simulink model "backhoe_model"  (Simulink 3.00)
settings: Solver=ode4  StartTime=0.0  StopTime=tfinal  FixedStep=T  RelTol=1e-3
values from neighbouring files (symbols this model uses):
  a1 = R(1,1)    [Jacobian.m]    (also in sub_static_vars.m = a(1))
  a2 = R(2,2)    [Jacobian.m]    (also in sub_static_vars.m = a(2))
  a3 = R(3,3)    [Jacobian.m]    (also in sub_static_vars.m = a(3))
  a4 = R(4,1)    [Jacobian.m]    (also in sub_static_vars.m = a(4))
  Ac = pi*(Dc.^2)/4    [cylinders.m]
  Ar = Ac-pi*(Dr.^2)/4    [cylinders.m]
  Cd = 2    [startup.m]
  dt = tfinal/N    (= 0.02)    [demo_trench.m]
  G1 = '0'    [sub_static_vars.m]    (also in symbolic_manip.m = G)
  G2 = char(G{2})    [sub_static_vars.m]    (also in symbolic_manip.m = G)
  G3 = char(G{3})    [sub_static_vars.m]    (also in symbolic_manip.m = G)
  G4 = char(G{4})    [sub_static_vars.m]    (also in symbolic_manip.m = G)
  Lcyl = [12.5*2 25 25.5 21.5]'    [cylinders.m]
  M11 = char(M{1})    [sub_static_vars.m]
  M12 = char(M{2})    [sub_static_vars.m]
  M13 = char(M{3})    [sub_static_vars.m]
  M14 = char(M{4})    [sub_static_vars.m]
  M21 = char(M{5})    [sub_static_vars.m]
  M22 = char(M{6})    [sub_static_vars.m]
  M23 = char(M{7})    [sub_static_vars.m]
  M24 = char(M{8})    [sub_static_vars.m]
  M31 = char(M{9})    [sub_static_vars.m]
  M32 = char(M{10})    [sub_static_vars.m]
  M33 = char(M{11})    [sub_static_vars.m]
  M34 = char(M{12})    [sub_static_vars.m]
  M41 = char(M{13})    [sub_static_vars.m]
  M42 = char(M{14})    [sub_static_vars.m]
  M43 = char(M{15})    [sub_static_vars.m]
  M44 = char(M{16})    [sub_static_vars.m]
  prelief = 2250    [backhoesim.m]
  pT = 0    [backhoesim.m]
  q0 = cyl_to_joint(yc0,R)    [backhoesim.m]
  qmax = cyl_to_joint([yclim(2,1) yclim(2,1) yclim(1,2) yclim(1,3) yclim(1,4)],R)    [backhoesim.m]    (also in demo_trench.m = [1.5708    1.0907    6.1403    6.5025])
  qmin = cyl_to_joint([yclim(1,1) yclim(1,1) yclim(2,2) yclim(2,3) yclim(2,4)],R)    [backhoesim.m]    (also in demo_trench.m = [-1.5708   -0.8529    3.6469    4.1089])
  QP = 33.11    [backhoesim.m]
  R1A = R(1,5)    [cyl_to_joint.m]    (also in dimensions.m = sqrt(R0N^2+(R01-RAN)^2); joint_to_cyl.m; SFr2taur.m; Sjoint_to_cyl.m)
  R1B = R(2,4)    [cyl_to_joint.m]    (also in dimensions.m = 35.875; joint_to_cyl.m; SFr2taur.m; Sjoint_to_cyl.m)
  R2C = R(2,3)    [cyl_to_joint.m]    (also in dimensions.m = 36; joint_to_cyl.m; SFr2taur.m; Sjoint_to_cyl.m)
  R2D = R(3,1)    [cyl_to_joint.m]    (also in dimensions.m = 9.875; joint_to_cyl.m; SFr2taur.m; Sjoint_to_cyl.m)
  R3F = R(3,5)-R(3,7)    [cyl_to_joint.m]    (also in dimensions.m = 4.5; joint_to_cyl.m; SFr2taur.m = R(3,8); Sjoint_to_cyl.m)
  R3G = R(4,2)    [cyl_to_joint.m]    (also in dimensions.m = 5.5; joint_to_cyl.m; SFr2taur.m; Sjoint_to_cyl.m)
  REF = R(3,6)    [cyl_to_joint.m]    (also in dimensions.m = 30.77; joint_to_cyl.m; SFr2taur.m; Sjoint_to_cyl.m)
  RFH = R(4,4)    [cyl_to_joint.m]    (also in dimensions.m = 9.5; joint_to_cyl.m; SFr2taur.m; Sjoint_to_cyl.m)
  RGH = R(4,5)    [cyl_to_joint.m]    (also in dimensions.m = 9.5; joint_to_cyl.m; SFr2taur.m; Sjoint_to_cyl.m)
  T = 0.001    [startup.m]
  T01A = R(1,12)    [cyl_to_joint.m]    (also in dimensions.m = atan(R0N/(R01-RAN)); joint_to_cyl.m; Sjoint_to_cyl.m)
  T12C = R(2,13)    [cyl_to_joint.m]    (also in dimensions.m = acos((R12^2+R2C^2-R1C^2)/(2*R12*R2C)); joint_to_cyl.m; Sjoint_to_cyl.m)
  T23D = acos((R23^2+R3D^2-R2D^2)/(2*R23*R3D))    [cyl_to_joint.m]    (also in dimensions.m; joint_to_cyl.m = R(3,14); SFr2taur.m = R(3,14); Sjoint_to_cyl.m = R(3,14))
  TB12 = R(2,12)    [cyl_to_joint.m]    (also in dimensions.m = acos((R1B^2+R12^2-R2B^2)/(2*R1B*R12)); joint_to_cyl.m; SFr2taur.m; Sjoint_to_cyl.m)
  TD23 = R(3,12)    [cyl_to_joint.m]    (also in dimensions.m = acos((R2D^2+R23^2-R3D^2)/(2*R2D*R23)); joint_to_cyl.m; SFr2taur.m; Sjoint_to_cyl.m)
  TDFE = R(3,13)    [cyl_to_joint.m]    (also in dimensions.m = acos((RDF^2+REF^2-RDE^2)/(2*RDF*REF)); joint_to_cyl.m; SFr2taur.m; Sjoint_to_cyl.m)
  TG34 = R(4,12)    [cyl_to_joint.m]    (also in dimensions.m = acos((R3G^2+R34^2-R4G^2)/(2*R3G*R34)); joint_to_cyl.m; SFr2taur.m; Sjoint_to_cyl.m)
  V1 = char(V{1})    [sub_static_vars.m]    (also in symbolic_manip.m = V)
  V2 = char(V{2})    [sub_static_vars.m]    (also in symbolic_manip.m = V)
  V3 = char(V{3})    [sub_static_vars.m]    (also in symbolic_manip.m = V)
  V4 = char(V{4})    [sub_static_vars.m]    (also in symbolic_manip.m = V)
  yc0 = [21.587 21.587 28.9 45.27 36.195]'    [backhoesim.m]
undefined symbols (not defined in the file or in its folder): Cc, Cr, den, K1, kd, Kr, num, pc0, pr0, td, wn, zeta
libraries: simulink3 x2
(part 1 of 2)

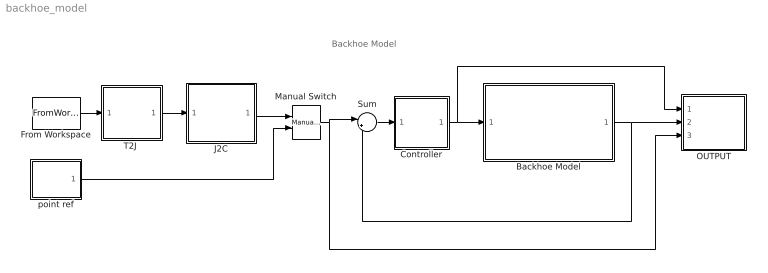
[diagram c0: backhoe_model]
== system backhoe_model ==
  note: Backhoe Model
  Backhoe Model : Subsystem
  Controller : Subsystem
  From Workspace : FromWorkspace  VariableName=traj  SampleTime=0  HoldFinalValue=off
  J2C : Subsystem
  Manual Switch : simulink3/Nonlinear/Manual Switch  sw=1  action=0
  OUTPUT : Subsystem
  Sum : Sum  Inputs=|+-  SaturateOnIntegerOverflow=on
  "T2J " : Subsystem
  point ref : Subsystem
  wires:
  Sum/1 -> Controller/1(e)
  Backhoe Model/1(yc_th) -> Sum/2, OUTPUT/2(yc_th)
  Controller/1(Us) -> Backhoe Model/1(Us), OUTPUT/1(Us)
  Manual Switch/1 -> Sum/1, OUTPUT/3(ycdes)
  J2C/1(ycdes) -> Manual Switch/1
  "T2J "/1(qdes) -> J2C/1(qdes)
  From Workspace/1 -> "T2J "/1(ybdes)
  point ref/1(ycdes) -> Manual Switch/2

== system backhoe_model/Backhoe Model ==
  note: Note: input voltages need to range between (3,9) [V]
  note: predicted position sensor measurements
  Us : Inport  Port=1  PortWidth=-1  SampleTime=-1  DataType=auto
  Backhoe Dynamics : Subsystem
  Hoses & Cylinders : Subsystem
  Mux : Mux  Inputs=2
  PVG32 Valve Bank : Subsystem
  Selector : Selector  Elements=[3 4 5]  InputPortWidth=5
  Subsystem : Subsystem
  Terminator5 : Terminator
  Terminator6 : Terminator
  pump flow rate : Constant  Value=QP
  soil wrench : Constant  Value=[0 0 0 0 0 0]
  tank pressure : Constant  Value=pT
  yc_th : Outport  Port=1
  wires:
  Backhoe Dynamics/3(yc) -> Hoses & Cylinders/3(yc), Selector/1
  Backhoe Dynamics/2(yed) -> Terminator5/1
  soil wrench/1 -> Backhoe Dynamics/2(We)
  [pcyl] -> PVG32 Valve Bank/2(pcyl)
  pump flow rate/1 -> PVG32 Valve Bank/3(QP)
  tank pressure/1 -> PVG32 Valve Bank/4(pT)
  Hoses & Cylinders/2(Fr) -> Backhoe Dynamics/1(Fr)
  Backhoe Dynamics/1(ye) -> Terminator6/1
  Us/1 -> PVG32 Valve Bank/1(Us)
  Selector/1 -> Mux/2
  Backhoe Dynamics/4(q1) -> Mux/1
  Hoses & Cylinders/1(pcyl) -> [pcyl], Subsystem/1(pcyl1)
  Mux/1 -> yc_th/1
  PVG32 Valve Bank/1(Qc) -> Hoses & Cylinders/1(Qc)
  PVG32 Valve Bank/2(Qr) -> Hoses & Cylinders/2(Qr)

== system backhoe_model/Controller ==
  note: Controller
  e : Inport  Port=1  PortWidth=-1  SampleTime=-1  DataType=auto
  Anti-deadband : Subsystem
  D-Gain : Gain  Gain=[0 0 0 0]  SaturateOnIntegerOverflow=on
  Derivative : Derivative
  I-Gain : Gain  Gain=[0 0 0 0]  SaturateOnIntegerOverflow=on
  Integrator : Integrator  ExternalReset=none  InitialConditionSource=internal  InitialCondition=0  LimitOutput=on  UpperSaturationLimit=1  LowerSaturationLimit=-1  ShowSaturationPort=off  ShowStatePort=off  AbsoluteTolerance=auto
  Manual Switch : simulink3/Nonlinear/Manual Switch  sw=1  action=0
  P-Gain : Gain  Gain=[0.8 0.8 0.8 0.8]  SaturateOnIntegerOverflow=on
  Standard : Subsystem
  Sum : Sum  Inputs=+++  SaturateOnIntegerOverflow=on
  voltage limits : Saturate  UpperLimit=9  LowerLimit=3
  Us : Outport  Port=1
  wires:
  e/1 -> P-Gain/1, I-Gain/1, D-Gain/1
  D-Gain/1 -> Derivative/1
  Integrator/1 -> Sum/2
  I-Gain/1 -> Integrator/1
  P-Gain/1 -> Sum/1
  Derivative/1 -> Sum/3
  Sum/1 -> Anti-deadband/1(us), Standard/1(us)
  Standard/1(Us) -> Manual Switch/1
  Manual Switch/1 -> voltage limits/1
  voltage limits/1 -> Us/1
  Anti-deadband/1(Us) -> Manual Switch/2

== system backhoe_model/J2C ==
  note: Joint Space -> Cylinder Space Transformation
  note: Swing Cylinders
  qdes : Inport  Port=1  PortWidth=-1  SampleTime=-1  DataType=auto
  Boom cylinder : Subsystem
  Bucket cylinder : Subsystem
  Demux : Demux  Outputs=4
  Mux : Mux  Inputs=4
  Stick cylinder : Subsystem
  overswing  protection : Saturate  UpperLimit=pi/3  LowerLimit=-pi/2
  ycdes : Outport  Port=1
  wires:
  qdes/1 -> Demux/1
  Mux/1 -> ycdes/1
  Demux/2 -> Boom cylinder/1(q2)
  Boom cylinder/1(yc3) -> Mux/2
  Demux/3 -> Stick cylinder/1(q3)
  Stick cylinder/1(yc4) -> Mux/3
  Demux/4 -> Bucket cylinder/1(q4)
  Bucket cylinder/1(yc5) -> Mux/4
  Demux/1 -> overswing  protection/1
  overswing  protection/1 -> Mux/1

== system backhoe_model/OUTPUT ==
  Us : Inport  Port=1  PortWidth=-1  SampleTime=-1  DataType=auto
  yc_th : Inport  Port=2  PortWidth=-1  SampleTime=-1  DataType=auto
  ycdes : Inport  Port=3  PortWidth=-1  SampleTime=-1  DataType=auto
  Clock : Clock
  Demux : Demux  Outputs=4
  Demux1 : Demux  Outputs=4
  Mux : Mux  Inputs=4
  Mux{1..4} (4 alike) : Mux  Inputs=2
  To Workspace : ToWorkspace  VariableName=data_th  SampleTime=-1  SaveFormat=Matrix
  Us1 : Scope
  yc : Scope  NumInputPorts=4
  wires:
  Mux/1 -> To Workspace/1
  Clock/1 -> Mux/1
  Us/1 -> Mux/2, Us1/1
  yc_th/1 -> Mux/3, Demux/1
  Mux1/1 -> yc/1
  Mux2/1 -> yc/2
  Mux3/1 -> yc/3
  Mux4/1 -> yc/4
  Demux1/1 -> Mux1/1
  Demux/1 -> Mux1/2
  Demux1/2 -> Mux2/1
  Demux/2 -> Mux2/2
  Demux1/3 -> Mux3/1
  Demux/3 -> Mux3/2
  Demux1/4 -> Mux4/1
  Demux/4 -> Mux4/2
  ycdes/1 -> Demux1/1, Mux/4

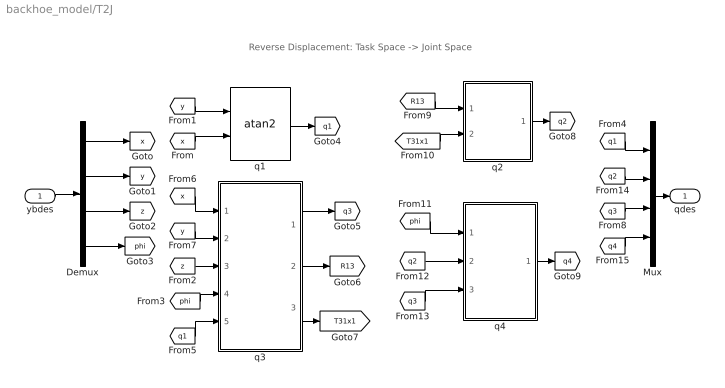
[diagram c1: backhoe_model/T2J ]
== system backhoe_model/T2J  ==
  note: Reverse Displacement: Task Space -> Joint Space
  ybdes : Inport  Port=1  PortWidth=-1  SampleTime=-1  DataType=auto
  Demux : Demux  Outputs=4
  Mux : Mux  Inputs=4
  q1 : Trigonometry  Operator=atan2  OutputSignalType=auto
  q2 : Subsystem
  q3 : Subsystem
  q4 : Subsystem
  qdes : Outport  Port=1
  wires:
  [x] -> q3/1(x)
  [y] -> q3/2(y)
  [z] -> q3/3(z)
  [phi] -> q3/4(phi)
  [q1] -> q3/5(q1)
  q3/1(q3) -> [q3]
  q3/2(R13) -> [R13]
  [y] -> q1/1
  q1/1 -> [q1]
  q3/3(T31x1) -> [T31x1]
  [R13] -> q2/1(R13)
  [T31x1] -> q2/2(T31x1)
  [q3] -> q4/3(q3)
  [q2] -> q4/2(q2)
  [phi] -> q4/1(phi)
  q2/1(q2) -> [q2]
  q4/1(q4) -> [q4]
  Mux/1 -> qdes/1
  [q1] -> Mux/1
  [q3] -> Mux/3
  [q2] -> Mux/2
  [q4] -> Mux/4
  ybdes/1 -> Demux/1
  Demux/1 -> [x]
  Demux/2 -> [y]
  Demux/3 -> [z]
  Demux/4 -> [phi]
  [x] -> q1/2

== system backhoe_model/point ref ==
  Boom : Sin  Amplitude=0  Frequency=1  Phase=0  SampleTime=0
  Bucket : Sin  Amplitude=0  Frequency=1  Phase=0  SampleTime=0
  Mux : Mux  Inputs=4
  Stick : Sin  Amplitude=0  Frequency=1  Phase=0  SampleTime=0
  Sum : Sum  Inputs=|++  SaturateOnIntegerOverflow=on
  Swing : Sin  Amplitude=0.3  Frequency=0.7  Phase=0  SampleTime=0
  initial cylinder lengths : Constant  Value=[q0(1) yc0(3) yc0(4) yc0(5)]
  ycdes : Outport  Port=1
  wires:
  Swing/1 -> Mux/1
  Boom/1 -> Mux/2
  Bucket/1 -> Mux/4
  Stick/1 -> Mux/3
  Mux/1 -> Sum/1
  initial cylinder lengths/1 -> Sum/2
  Sum/1 -> ycdes/1

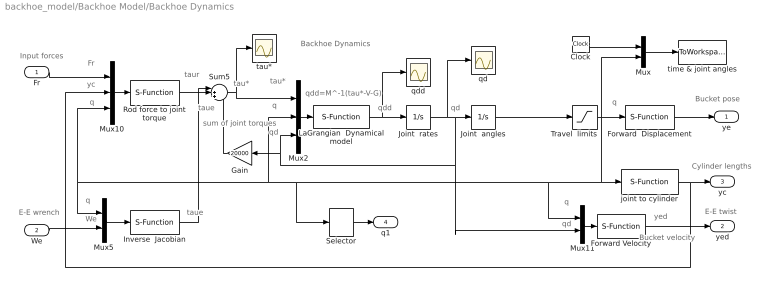
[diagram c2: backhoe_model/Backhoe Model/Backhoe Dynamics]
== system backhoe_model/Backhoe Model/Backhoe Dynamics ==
  note: taur
  note: tau*
  note: qdd
  note: qd
  note: qdd=M^-1(tau*-V-G)
  note: q
  note: q
  note: taue
  note: taue
  note: Bucket velocity
  note: yed
  note: qd
  note: q
  note: qd
  note: Fr
  note: q
  note: tau*
  note: sum of joint torques
  note: yc
  note: q
  note: We
  note: Backhoe Dynamics
  note: E-E wrench
  note: Input forces
  note: Bucket pose
  note: Cylinder lengths
  note: E-E twist
  Fr : Inport  Port=1  PortWidth=-1  SampleTime=-1  DataType=auto
  We : Inport  Port=2  PortWidth=-1  SampleTime=-1  DataType=auto
  Clock : Clock
  Forward Velocity : S-Function  FunctionName=SFvel  Parameters=R  PortCounts=[]  SFunctionModules=''
  Forward  Displacement : S-Function  FunctionName=SFdisp  Parameters=a  PortCounts=[]  SFunctionModules=''
  Gain : Gain  Orientation=left  Gain=20000  SaturateOnIntegerOverflow=on
  Inverse  Jacobian : S-Function  FunctionName=SRtorque  Parameters=R  PortCounts=[]  SFunctionModules=''
  Joint  angles : Integrator  ExternalReset=none  InitialConditionSource=internal  InitialCondition=q0  LimitOutput=off  UpperSaturationLimit=inf  LowerSaturationLimit=-inf  ShowSaturationPort=off  ShowStatePort=off  AbsoluteTolerance=auto
  Joint  rates : Integrator  ExternalReset=none  InitialConditionSource=internal  InitialCondition=0  LimitOutput=off  UpperSaturationLimit=inf  LowerSaturationLimit=-inf  ShowSaturationPort=off  ShowStatePort=off  AbsoluteTolerance=auto
  LaGrangian  Dynamical model : S-Function  FunctionName=SLaGrange  Parameters=M11,M12,M13,M14,M21,M22,M23,M24,M31,M32,M33,M34,M41,M42,M43,M44,V1,V2,V3,V4,G1,G2,G3,G4  PortCounts=[]  SFunctionModules=''
  Mux : Mux  Inputs=2
  Mux10 : Mux  Inputs=3
  Mux11 : Mux  Inputs=2
  Mux2 : Mux  Inputs=3
  Mux5 : Mux  Inputs=2
  Rod force to joint torque : S-Function  FunctionName=SFr2taur  Parameters=R  PortCounts=[]  SFunctionModules=''
  Selector : Selector  Elements=1  InputPortWidth=4
  Sum5 : Sum  Inputs=|++-  SaturateOnIntegerOverflow=on
  Travel  limits : Saturate  UpperLimit=qmax  LowerLimit=qmin
  joint to cylinder : S-Function  FunctionName=Sjoint_to_cyl  Parameters=R, yc0  PortCounts=[]  SFunctionModules=''
  qd : Scope
  qdd : Scope
  tau* : Scope
  time & joint angles : ToWorkspace  VariableName=tq  SampleTime=-1  SaveFormat=Matrix
  ye : Outport  Port=1
  yed : Outport  Port=2
  yc : Outport  Port=3
  q1 : Outport  Port=4
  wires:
  Mux2/1 -> LaGrangian  Dynamical model/1
  Mux10/1 -> Rod force to joint torque/1
  Rod force to joint torque/1 -> Sum5/1
  Mux5/1 -> Inverse  Jacobian/1
  Inverse  Jacobian/1 -> Sum5/2
  We/1 -> Mux5/2
  Selector/1 -> q1/1
  Sum5/1 -> Mux2/1, tau*/1
  Fr/1 -> Mux10/1
  LaGrangian  Dynamical model/1 -> Joint  rates/1, qdd/1
  Joint  rates/1 -> Mux11/2, Mux2/3, Gain/1, Joint  angles/1, qd/1
  Clock/1 -> Mux/1
  Travel  limits/1 -> Forward  Displacement/1, Mux11/1, Mux2/2, Mux5/1, Mux10/3, Selector/1, joint to cylinder/1, Mux/2
  Mux11/1 -> Forward Velocity/1
  joint to cylinder/1 -> yc/1, Mux10/2
  Forward Velocity/1 -> yed/1
  Forward  Displacement/1 -> ye/1
  Mux/1 -> time & joint angles/1
  Joint  angles/1 -> Travel  limits/1
  Gain/1 -> Sum5/3

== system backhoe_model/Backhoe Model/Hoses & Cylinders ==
  note: DVc
  note: DVr
  note: pc
  note: cap pressures
  note: pr
  note: rod pressures
  note: pressure forces on rods
  note: yc
  note: yc
  note: Hoses and Cylinders
  Qc : Inport  Port=1  PortWidth=-1  SampleTime=-1  DataType=auto
  Qr : Inport  Port=2  PortWidth=-1  SampleTime=-1  DataType=auto
  yc : Inport  Port=3  PortWidth=-1  SampleTime=-1  DataType=auto
  Cap areas : Gain  Gain=Ac  SaturateOnIntegerOverflow=on
  Cap-side compressible  volume : S-Function  FunctionName=SCcap  Parameters=Ac,Cc,yc0,pc0  PortCounts=[]  SFunctionModules=''
  DVcDVr : Scope  NumInputPorts=2
  Fr1 : Scope
  Integrator : Integrator  ExternalReset=none  InitialConditionSource=internal  InitialCondition=0  LimitOutput=on  UpperSaturationLimit=Lcyl.*Ac  LowerSaturationLimit=-Lcyl.*Ac  ShowSaturationPort=off  ShowStatePort=off  AbsoluteTolerance=auto
  Integrator1 : Integrator  ExternalReset=none  InitialConditionSource=internal  InitialCondition=0  LimitOutput=on  UpperSaturationLimit=Lcyl.*Ar  LowerSaturationLimit=-Lcyl.*Ar  ShowSaturationPort=off  ShowStatePort=off  AbsoluteTolerance=auto
  Mux : Mux  Inputs=2
  Mux7 : Mux  Inputs=2
  Mux8 : Mux  Inputs=2
  QcycQr : Scope  NumInputPorts=3
  Rod areas : Gain  Gain=Ar  SaturateOnIntegerOverflow=on
  Rod-side compressible volume : S-Function  FunctionName=SCrod  Parameters=Ar,Cr,yc0,pr0  PortCounts=[]  SFunctionModules=''
  Sum4 : Sum  Inputs=+|-  SaturateOnIntegerOverflow=on
  anti-cavitation : Saturate  UpperLimit=prelief  LowerLimit=0
  anti-cavitation1 : Saturate  UpperLimit=prelief  LowerLimit=0
  pcyl : Outport  Port=1
  Fr : Outport  Port=2
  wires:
  Cap-side compressible  volume/1 -> anti-cavitation/1
  Rod-side compressible volume/1 -> anti-cavitation1/1
  Cap areas/1 -> Sum4/1
  Mux/1 -> pcyl/1
  anti-cavitation/1 -> Cap areas/1, Mux/1
  anti-cavitation1/1 -> Rod areas/1, Mux/2
  yc/1 -> Mux8/2, Mux7/2, QcycQr/2
  Rod areas/1 -> Sum4/2
  Qr/1 -> Integrator1/1, QcycQr/3
  Qc/1 -> Integrator/1, QcycQr/1
  Sum4/1 -> Fr/1, Fr1/1
  Mux7/1 -> Cap-side compressible  volume/1
  Mux8/1 -> Rod-side compressible volume/1
  Integrator/1 -> Mux7/1, DVcDVr/1
  Integrator1/1 -> Mux8/1, DVcDVr/2

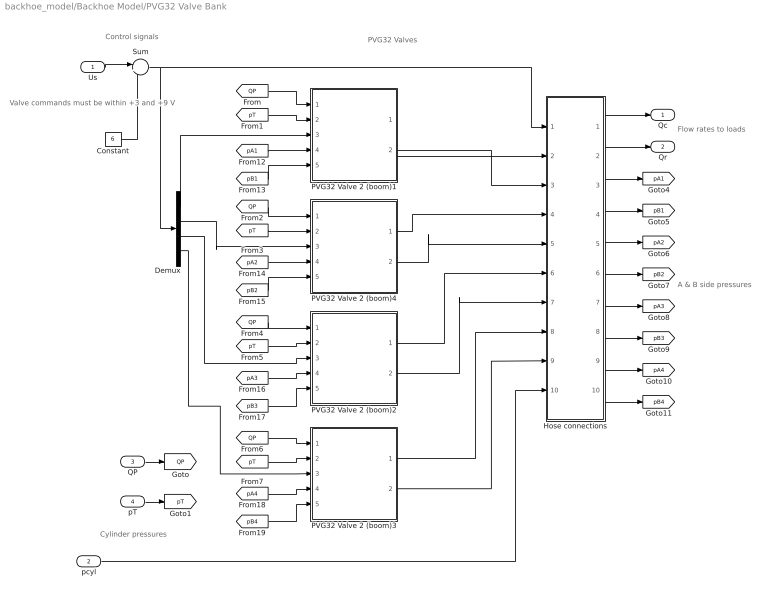
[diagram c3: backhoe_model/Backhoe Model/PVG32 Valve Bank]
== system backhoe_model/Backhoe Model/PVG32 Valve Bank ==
  note: Flow rates to loads
  note: Control signals
  note: PVG32 Valves
  note: Cylinder pressures
  note: A & B side pressures
  note: Valve commands must be within +3 and +9 V
  Us : Inport  Port=1  PortWidth=-1  SampleTime=-1  DataType=auto
  pcyl : Inport  Port=2  PortWidth=-1  SampleTime=-1  DataType=auto
  QP : Inport  Port=3  PortWidth=-1  SampleTime=-1  DataType=auto
  pT : Inport  Port=4  PortWidth=-1  SampleTime=-1  DataType=auto
  Constant : Constant  Value=6
  Demux : Demux  Outputs=4
  Hose connections : Subsystem
  PVG32 Valve 2 (boom)1 : Subsystem
  PVG32 Valve 2 (boom)2 : Subsystem
  PVG32 Valve 2 (boom)3 : Subsystem
  PVG32 Valve 2 (boom)4 : Subsystem
  Sum : Sum  Inputs=|+-  SaturateOnIntegerOverflow=on
  Qc : Outport  Port=1
  Qr : Outport  Port=2
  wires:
  Hose connections/1(Qc) -> Qc/1
  Hose connections/2(Qr) -> Qr/1
  Hose connections/3(pA1) -> [pA1]
  Hose connections/4(pB1) -> [pB1]
  Hose connections/5(pA2) -> [pA2]
  Hose connections/6(pB2) -> [pB2]
  Hose connections/7(pA3) -> [pA3]
  Hose connections/8(pB3) -> [pB3]
  Hose connections/9(pA4) -> [pA4]
  Hose connections/10(pB4) -> [pB4]
  pcyl/1 -> Hose connections/10(pcyl)
  Demux/1 -> PVG32 Valve 2 (boom)1/3(Us)
  [QP] -> PVG32 Valve 2 (boom)1/1(QP)
  [pT] -> PVG32 Valve 2 (boom)1/2(pT)
  [pA1] -> PVG32 Valve 2 (boom)1/4(pA)
  [pB1] -> PVG32 Valve 2 (boom)1/5(pB)
  Demux/2 -> PVG32 Valve 2 (boom)4/3(Us)
  [pT] -> PVG32 Valve 2 (boom)4/2(pT)
  [QP] -> PVG32 Valve 2 (boom)4/1(QP)
  Demux/3 -> PVG32 Valve 2 (boom)2/3(Us)
  [pA2] -> PVG32 Valve 2 (boom)4/4(pA)
  [pB2] -> PVG32 Valve 2 (boom)4/5(pB)
  [pT] -> PVG32 Valve 2 (boom)2/2(pT)
  [QP] -> PVG32 Valve 2 (boom)2/1(QP)
  [pA3] -> PVG32 Valve 2 (boom)2/4(pA)
  [pB3] -> PVG32 Valve 2 (boom)2/5(pB)
  Demux/4 -> PVG32 Valve 2 (boom)3/3(Us)
  QP/1 -> [QP]
  pT/1 -> [pT]
  [QP] -> PVG32 Valve 2 (boom)3/1(QP)
  [pT] -> PVG32 Valve 2 (boom)3/2(pT)
  [pA4] -> PVG32 Valve 2 (boom)3/4(pA)
  [pB4] -> PVG32 Valve 2 (boom)3/5(pB)
  PVG32 Valve 2 (boom)1/1(QA) -> Hose connections/2(QA1)
  PVG32 Valve 2 (boom)1/2(QB) -> Hose connections/3(QB1)
  PVG32 Valve 2 (boom)4/1(QA) -> Hose connections/4(QA2)
  PVG32 Valve 2 (boom)4/2(QB) -> Hose connections/5(QB2)
  PVG32 Valve 2 (boom)2/1(QA) -> Hose connections/6(QA3)
  PVG32 Valve 2 (boom)2/2(QB) -> Hose connections/7(QB3)
  PVG32 Valve 2 (boom)3/1(QA) -> Hose connections/8(QA4)
  PVG32 Valve 2 (boom)3/2(QB) -> Hose connections/9(QB4)
  Us/1 -> Sum/1
  Constant/1 -> Sum/2
  Sum/1 -> Demux/1, Hose connections/1(Us)

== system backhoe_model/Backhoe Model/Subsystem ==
  pcyl1 : Inport  Port=1  PortWidth=-1  SampleTime=-1  DataType=auto
  Selector : Selector  Elements=[1 5]  InputPortWidth=8
  Selector1 : Selector  Elements=[2 6]  InputPortWidth=8
  Selector2 : Selector  Elements=[3 7]  InputPortWidth=8
  Selector3 : Selector  Elements=[4 8]  InputPortWidth=8
  To Workspace : ToWorkspace  VariableName=pcyl  SampleTime=-1  SaveFormat=Matrix
  pcyl : Scope  NumInputPorts=4
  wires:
  pcyl1/1 -> To Workspace/1, Selector3/1, Selector2/1, Selector/1, Selector1/1
  Selector/1 -> pcyl/1
  Selector1/1 -> pcyl/2
  Selector2/1 -> pcyl/3
  Selector3/1 -> pcyl/4

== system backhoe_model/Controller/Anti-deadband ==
  us : Inport  Port=1  PortWidth=-1  SampleTime=-1  DataType=auto
  Demux : Demux  Outputs=4
  Look-Up Table{,1..3} (4 alike) : Lookup  InputValues=[-1 0.02 0.02 1]  OutputValues=[3 5.45 6.55 9]
  Mux : Mux  Inputs=4
  Saturation : Saturate  UpperLimit=9  LowerLimit=3
  Us : Outport  Port=1
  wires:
  Demux/1 -> Look-Up Table/1
  Demux/2 -> Look-Up Table1/1
  Demux/3 -> Look-Up Table2/1
  Demux/4 -> Look-Up Table3/1
  Look-Up Table/1 -> Mux/1
  us/1 -> Demux/1
  Mux/1 -> Saturation/1
  Saturation/1 -> Us/1
  Look-Up Table1/1 -> Mux/2
  Look-Up Table2/1 -> Mux/3
  Look-Up Table3/1 -> Mux/4

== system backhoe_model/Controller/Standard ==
  us : Inport  Port=1  PortWidth=-1  SampleTime=-1  DataType=auto
  Gain : Gain  Gain=[10 3 3 1.5]  SaturateOnIntegerOverflow=on
  Sum1 : Sum  Inputs=|++  SaturateOnIntegerOverflow=on
  neutral : Constant  Value=6
  Us : Outport  Port=1
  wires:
  us/1 -> Gain/1
  neutral/1 -> Sum1/2
  Gain/1 -> Sum1/1
  Sum1/1 -> Us/1

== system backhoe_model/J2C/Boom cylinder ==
  q2 : Inport  Port=1  PortWidth=-1  SampleTime=-1  DataType=auto
  Constant : Constant  Value=pi
  Constant1 : Constant  Value=T01A
  Constant2 : Constant  Value=TB12
  CosineLawB : Subsystem
  Sum : Sum  Inputs=+---  SaturateOnIntegerOverflow=on
  yc3 : Outport  Port=1
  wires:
  Constant/1 -> Sum/1
  Constant1/1 -> Sum/2
  Sum/1 -> CosineLawB/1(TA1B)
  CosineLawB/1(yc3) -> yc3/1
  q2/1 -> Sum/3
  Constant2/1 -> Sum/4

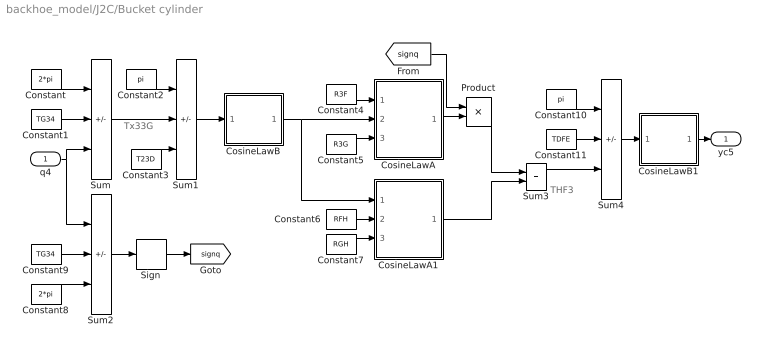
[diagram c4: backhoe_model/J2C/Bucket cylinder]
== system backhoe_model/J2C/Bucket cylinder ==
  note: Tx33G
  note: THF3
  q4 : Inport  Port=1  PortWidth=-1  SampleTime=-1  DataType=auto
  Constant : Constant  Value=2*pi
  Constant1 : Constant  Value=TG34
  Constant10 : Constant  Value=pi
  Constant11 : Constant  Value=TDFE
  Constant2 : Constant  Value=pi
  Constant3 : Constant  Value=T23D
  Constant4 : Constant  Value=R3F
  Constant5 : Constant  Value=R3G
  Constant6 : Constant  Value=RFH
  Constant7 : Constant  Value=RGH
  Constant8 : Constant  Value=2*pi
  Constant9 : Constant  Value=TG34
  CosineLawA : Subsystem
  CosineLawA1 : Subsystem
  CosineLawB : Subsystem
  CosineLawB1 : Subsystem
  Product : Product  Inputs=2  SaturateOnIntegerOverflow=on
  Sign : Signum
  Sum : Sum  Inputs=+--  SaturateOnIntegerOverflow=on
  Sum1 : Sum  Inputs=+-+  SaturateOnIntegerOverflow=on
  Sum2 : Sum  Inputs=++-  SaturateOnIntegerOverflow=on
  Sum3 : Sum  Inputs=++  SaturateOnIntegerOverflow=on
  Sum4 : Sum  Inputs=+--  SaturateOnIntegerOverflow=on
  yc5 : Outport  Port=1
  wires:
  Constant/1 -> Sum/1
  Constant1/1 -> Sum/2
  Sum/1 -> Sum1/2
  Constant2/1 -> Sum1/1
  Sum1/1 -> CosineLawB/1(TG3F)
  CosineLawB/1(rFG) -> CosineLawA/2(r2), CosineLawA1/1(r1)
  Constant4/1 -> CosineLawA/1(r1)
  Constant5/1 -> CosineLawA/3(r3)
  Constant6/1 -> CosineLawA1/2(r2)
  Constant7/1 -> CosineLawA1/3(r3)
  Constant9/1 -> Sum2/2
  Sum2/1 -> Sign/1
  [signq] -> Product/1
  CosineLawA/1(T3FG) -> Product/2
  Sign/1 -> [signq]
  Product/1 -> Sum3/1
  CosineLawA1/1(THFG) -> Sum3/2
  Constant10/1 -> Sum4/1
  Constant11/1 -> Sum4/2
  Sum4/1 -> CosineLawB1/1(TEFH)
  CosineLawB1/1(yc5) -> yc5/1
  q4/1 -> Sum2/1, Sum/3
  Constant3/1 -> Sum1/3
  Sum3/1 -> Sum4/3
  Constant8/1 -> Sum2/3

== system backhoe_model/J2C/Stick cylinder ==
  q3 : Inport  Port=1  PortWidth=-1  SampleTime=-1  DataType=auto
  Constant : Constant  Value=pi
  Constant1 : Constant  Value=TD23
  Constant2 : Constant  Value=T12C
  CosineLawB : Subsystem
  Sum : Sum  Inputs=+---  SaturateOnIntegerOverflow=on
  yc4 : Outport  Port=1
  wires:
  Constant/1 -> Sum/1
  Constant1/1 -> Sum/2
  Sum/1 -> CosineLawB/1(TC2D)
  CosineLawB/1(yc4) -> yc4/1
  q3/1 -> Sum/3
  Constant2/1 -> Sum/4

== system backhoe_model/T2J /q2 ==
  note: T213
  R13 : Inport  Port=1  PortWidth=-1  SampleTime=-1  DataType=auto
  T31x1 : Inport  Port=2  PortWidth=-1  SampleTime=-1  DataType=auto
  CosineLawA : Subsystem
  Sum : Sum  Inputs=|++  SaturateOnIntegerOverflow=on
  a2 : Constant  Value=a2
  a3 : Constant  Value=a3
  q2 : Outport  Port=1
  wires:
  a2/1 -> CosineLawA/1(r1)
  a3/1 -> CosineLawA/3(r3)
  CosineLawA/1(theta) -> Sum/1
  Sum/1 -> q2/1
  R13/1 -> CosineLawA/2(r2)
  T31x1/1 -> Sum/2

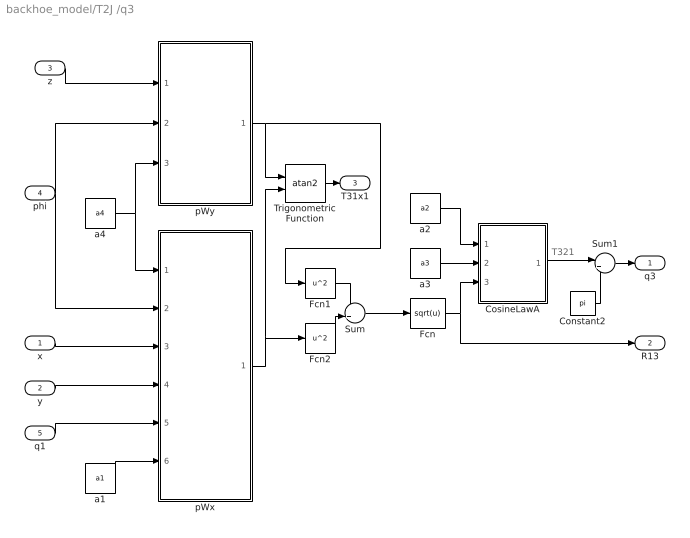
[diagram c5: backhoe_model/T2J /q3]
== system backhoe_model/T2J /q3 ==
  note: T321
  x : Inport  Port=1  PortWidth=-1  SampleTime=-1  DataType=auto
  y : Inport  Port=2  PortWidth=-1  SampleTime=-1  DataType=auto
  z : Inport  Port=3  PortWidth=-1  SampleTime=-1  DataType=auto
  phi : Inport  Port=4  PortWidth=-1  SampleTime=-1  DataType=auto
  q1 : Inport  Port=5  PortWidth=-1  SampleTime=-1  DataType=auto
  Constant2 : Constant  Value=pi
  CosineLawA : Subsystem
  Fcn : Fcn  Expr=sqrt(u)
  Fcn1 : Fcn  Expr=u^2
  Fcn2 : Fcn  Expr=u^2
  Sum : Sum  Inputs=++  SaturateOnIntegerOverflow=on
  Sum1 : Sum  Inputs=|++  SaturateOnIntegerOverflow=on
  Trigonometric Function : Trigonometry  Operator=atan2  OutputSignalType=auto
  a1 : Constant  Value=a1
  a2 : Constant  Value=a2
  a3 : Constant  Value=a3
  a4 : Constant  Value=a4
  pWx : Subsystem
  pWy : Subsystem
  q3 : Outport  Port=1
  R13 : Outport  Port=2
  T31x1 : Outport  Port=3
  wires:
  a1/1 -> pWx/6(a1)
  q1/1 -> pWx/5(q1)
  y/1 -> pWx/4(y)
  x/1 -> pWx/3(x)
  a4/1 -> pWx/1(a4), pWy/3(a4)
  z/1 -> pWy/1(z)
  phi/1 -> pWx/2(phi), pWy/2(phi)
  pWy/1(pWy) -> Fcn1/1, Trigonometric Function/1
  Trigonometric Function/1 -> T31x1/1
  Fcn1/1 -> Sum/1
  Fcn2/1 -> Sum/2
  Sum/1 -> Fcn/1
  a3/1 -> CosineLawA/2(r2)
  a2/1 -> CosineLawA/1(r1)
  Fcn/1 -> CosineLawA/3(r3), R13/1
  Sum1/1 -> q3/1
  Constant2/1 -> Sum1/2
  CosineLawA/1(theta) -> Sum1/1
  pWx/1(pWx) -> Fcn2/1, Trigonometric Function/2

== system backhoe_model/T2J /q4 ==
  phi : Inport  Port=1  PortWidth=-1  SampleTime=-1  DataType=auto
  q2 : Inport  Port=2  PortWidth=-1  SampleTime=-1  DataType=auto
  q3 : Inport  Port=3  PortWidth=-1  SampleTime=-1  DataType=auto
  Constant : Constant  Value=3*pi
  Sum : Sum  Inputs=+--+  SaturateOnIntegerOverflow=on
  q4 : Outport  Port=1
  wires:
  phi/1 -> Sum/1
  q2/1 -> Sum/2
  Sum/1 -> q4/1
  q3/1 -> Sum/3
  Constant/1 -> Sum/4

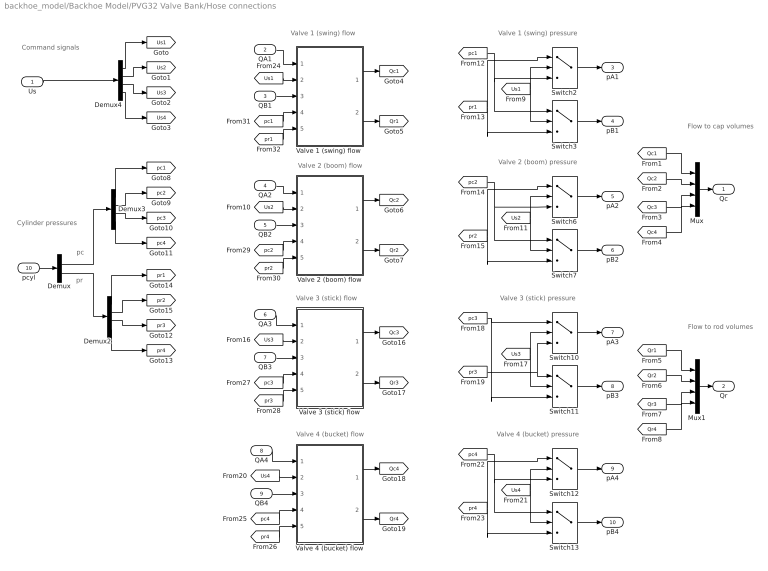
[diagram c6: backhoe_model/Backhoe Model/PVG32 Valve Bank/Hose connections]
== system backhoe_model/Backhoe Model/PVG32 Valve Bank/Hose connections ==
  note: pc
  note: pr
  note: Valve 1 (swing) flow
  note: Valve 1 (swing) pressure
  note: Valve 2 (boom) pressure
  note: Valve 3 (stick) flow
  note: Valve 3 (stick) pressure
  note: Valve 4 (bucket) flow
  note: Valve 4 (bucket) pressure
  note: Command signals
  note: Cylinder pressures
  note: Flow to rod volumes
  note: Flow to cap volumes
  note: Valve 2 (boom) flow
  Us : Inport  Port=1  PortWidth=-1  SampleTime=-1  DataType=auto
  QA1 : Inport  Port=2  PortWidth=-1  SampleTime=-1  DataType=auto
  QB1 : Inport  Port=3  PortWidth=-1  SampleTime=-1  DataType=auto
  QA2 : Inport  Port=4  PortWidth=-1  SampleTime=-1  DataType=auto
  QB2 : Inport  Port=5  PortWidth=-1  SampleTime=-1  DataType=auto
  QA3 : Inport  Port=6  PortWidth=-1  SampleTime=-1  DataType=auto
  QB3 : Inport  Port=7  PortWidth=-1  SampleTime=-1  DataType=auto
  QA4 : Inport  Port=8  PortWidth=-1  SampleTime=-1  DataType=auto
  QB4 : Inport  Port=9  PortWidth=-1  SampleTime=-1  DataType=auto
  pcyl : Inport  Port=10  PortWidth=-1  SampleTime=-1  DataType=auto
  Demux : Demux  Outputs=2
  Demux2 : Demux  Outputs=4
  Demux3 : Demux  Outputs=4
  Demux4 : Demux  Outputs=4
  Mux : Mux  Inputs=4
  Mux1 : Mux  Inputs=4
  Switch{2..3,6..7,10..13} (8 alike) : Switch  Threshold=0
  "Valve 1 (swing) flow " : Subsystem
  Valve 2 (boom) flow : Subsystem
  Valve 3 (stick) flow : Subsystem
  Valve 4 (bucket) flow : Subsystem
  Qc : Outport  Port=1
  Qr : Outport  Port=2
  pA1 : Outport  Port=3
  pB1 : Outport  Port=4
  pA2 : Outport  Port=5
  pB2 : Outport  Port=6
  pA3 : Outport  Port=7
  pB3 : Outport  Port=8
  pA4 : Outport  Port=9
  pB4 : Outport  Port=10
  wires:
  [Us1] -> Switch2/2, Switch3/2
  Switch2/1 -> pA1/1
  Switch3/1 -> pB1/1
  Demux3/1 -> [pc1]
  Demux3/2 -> [pc2]
  Demux3/3 -> [pc3]
  Demux3/4 -> [pc4]
  Demux2/1 -> [pr1]
  Demux2/2 -> [pr2]
  Demux2/3 -> [pr3]
  Demux2/4 -> [pr4]
  Demux4/1 -> [Us1]
  Demux4/2 -> [Us2]
  Demux4/3 -> [Us3]
  Demux4/4 -> [Us4]
  pcyl/1 -> Demux/1
  [pc1] -> Switch2/3, Switch3/1
  [pr1] -> Switch2/1, Switch3/3
  Demux/2 -> Demux2/1
  Demux/1 -> Demux3/1
  [Qc1] -> Mux/1
  [Qc2] -> Mux/2
  [Qc3] -> Mux/3
  [Qc4] -> Mux/4
  [Qr1] -> Mux1/1
  [Qr2] -> Mux1/2
  [Qr3] -> Mux1/3
  [Qr4] -> Mux1/4
  Mux/1 -> Qc/1
  Mux1/1 -> Qr/1
  Switch13/1 -> pB4/1
  Switch12/1 -> pA4/1
  [Us4] -> Switch12/2, Switch13/2
  [pc4] -> Switch12/3, Switch13/1
  [pr4] -> Switch13/3, Switch12/1
  Valve 4 (bucket) flow/1(Qc) -> [Qc4]
  Valve 4 (bucket) flow/2(Qr) -> [Qr4]
  QB4/1 -> Valve 4 (bucket) flow/3(QB)
  [Us4] -> Valve 4 (bucket) flow/2(Us)
  QA4/1 -> Valve 4 (bucket) flow/1(QA)
  [pc4] -> Valve 4 (bucket) flow/4(pc4)
  [pr4] -> Valve 4 (bucket) flow/5(pr4)
  [pr1] -> "Valve 1 (swing) flow "/5(pr1)
  [pc1] -> "Valve 1 (swing) flow "/4(pc1)
  QB1/1 -> "Valve 1 (swing) flow "/3(QB)
  [Us1] -> "Valve 1 (swing) flow "/2(Us)
  QA1/1 -> "Valve 1 (swing) flow "/1(QA)
  "Valve 1 (swing) flow "/1(Qc) -> [Qc1]
  "Valve 1 (swing) flow "/2(Qr) -> [Qr1]
  [Us2] -> Switch6/2, Switch7/2
  Switch6/1 -> pA2/1
  Switch7/1 -> pB2/1
  [pc2] -> Switch6/3, Switch7/1
  [pr2] -> Switch6/1, Switch7/3
  [pc2] -> Valve 2 (boom) flow/4(pc2)
  [pr2] -> Valve 2 (boom) flow/5(pr2)
  Valve 2 (boom) flow/1(Qc) -> [Qc2]
  Valve 2 (boom) flow/2(Qr) -> [Qr2]
  [Us2] -> Valve 2 (boom) flow/2(Us)
  QA2/1 -> Valve 2 (boom) flow/1(QA)
  QB2/1 -> Valve 2 (boom) flow/3(QB)
  Switch11/1 -> pB3/1
  Switch10/1 -> pA3/1
  [pr3] -> Switch11/1, Switch10/3
  [pc3] -> Switch10/1, Switch11/3
  [Us3] -> Switch10/2, Switch11/2
  Valve 3 (stick) flow/2(Qr) -> [Qr3]
  Valve 3 (stick) flow/1(Qc) -> [Qc3]
  [Us3] -> Valve 3 (stick) flow/2(Us)
  QA3/1 -> Valve 3 (stick) flow/1(QA)
  QB3/1 -> Valve 3 (stick) flow/3(QB)
  [pc3] -> Valve 3 (stick) flow/4(pc3)
  [pr3] -> Valve 3 (stick) flow/5(pr3)
  Us/1 -> Demux4/1

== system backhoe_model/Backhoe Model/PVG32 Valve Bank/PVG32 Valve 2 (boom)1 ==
  note: flow to load
  note: flow through relief valve
  QP : Inport  Port=1  PortWidth=-1  SampleTime=-1  DataType=auto
  pT : Inport  Port=2  PortWidth=-1  SampleTime=-1  DataType=auto
  Us : Inport  Port=3  PortWidth=-1  SampleTime=-1  DataType=auto
  pA : Inport  Port=4  PortWidth=-1  SampleTime=-1  DataType=auto
  pB : Inport  Port=5  PortWidth=-1  SampleTime=-1  DataType=auto
  Crossover relief : Subsystem  Orientation=left
  Dead Zone : DeadZone  LowerValue=-.5  UpperValue=.5
  Flow direction : Subsystem
  Input Averaging : Subsystem
  Product : Product  Inputs=2  SaturateOnIntegerOverflow=on
  SS gain : Subsystem
  Sum : Sum  Inputs=|+-  SaturateOnIntegerOverflow=on
  Terminator : Terminator
  Terminator2 : Terminator
  Time  Delay : TransportDelay  DelayTime=td  InitialInput=0  BufferSize=2048
  Valve dynamics : TransferFcn  Numerator=num  Denominator=den
  pump limits : Saturate  UpperLimit=QP  LowerLimit=-QP
  QA : Outport  Port=1
  QB : Outport  Port=2
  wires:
  pB/1 -> Flow direction/4(pB)
  pA/1 -> Flow direction/3(pA)
  pT/1 -> Terminator2/1
  Time  Delay/1 -> Valve dynamics/1
  Us/1 -> Dead Zone/1
  Dead Zone/1 -> Time  Delay/1, Flow direction/1(Us), Input Averaging/1(Us)
  Valve dynamics/1 -> Product/1
  Input Averaging/1(Ubar) -> SS gain/1(Ubar)
  SS gain/1(Kv) -> Product/2
  Product/1 -> Sum/1, Crossover relief/3(Q)
  Crossover relief/1(Qrelief) -> Sum/2
  QP/1 -> Terminator/1
  Sum/1 -> pump limits/1
  Flow direction/1(QA) -> QA/1
  Flow direction/2(QB) -> QB/1
  Flow direction/4(pR) -> Crossover relief/1(pR)
  Flow direction/3(pL) -> Crossover relief/2(pL)
  pump limits/1 -> Flow direction/2(Q)

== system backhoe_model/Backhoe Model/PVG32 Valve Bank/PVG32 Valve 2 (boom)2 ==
  note: flow to load
  note: flow through relief valve
  QP : Inport  Port=1  PortWidth=-1  SampleTime=-1  DataType=auto
  pT : Inport  Port=2  PortWidth=-1  SampleTime=-1  DataType=auto
  Us : Inport  Port=3  PortWidth=-1  SampleTime=-1  DataType=auto
  pA : Inport  Port=4  PortWidth=-1  SampleTime=-1  DataType=auto
  pB : Inport  Port=5  PortWidth=-1  SampleTime=-1  DataType=auto
  Crossover relief : Subsystem  Orientation=left
  Dead Zone : DeadZone  LowerValue=-.5  UpperValue=.5
  Flow direction : Subsystem
  Input Averaging : Subsystem
  Product : Product  Inputs=2  SaturateOnIntegerOverflow=on
  SS gain : Subsystem
  Sum : Sum  Inputs=|+-  SaturateOnIntegerOverflow=on
  Terminator : Terminator
  Terminator2 : Terminator
  Time  Delay : TransportDelay  DelayTime=td  InitialInput=0  BufferSize=2048
  Valve dynamics : TransferFcn  Numerator=num  Denominator=den
  pump limits : Saturate  UpperLimit=QP  LowerLimit=-QP
  QA : Outport  Port=1
  QB : Outport  Port=2
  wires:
  pB/1 -> Flow direction/4(pB)
  pA/1 -> Flow direction/3(pA)
  pT/1 -> Terminator2/1
  Time  Delay/1 -> Valve dynamics/1
  Us/1 -> Dead Zone/1
  Dead Zone/1 -> Time  Delay/1, Flow direction/1(Us), Input Averaging/1(Us)
  Valve dynamics/1 -> Product/1
  Input Averaging/1(Ubar) -> SS gain/1(Ubar)
  SS gain/1(Kv) -> Product/2
  Product/1 -> Sum/1, Crossover relief/3(Q)
  Crossover relief/1(Qrelief) -> Sum/2
  QP/1 -> Terminator/1
  Sum/1 -> pump limits/1
  Flow direction/1(QA) -> QA/1
  Flow direction/2(QB) -> QB/1
  Flow direction/4(pR) -> Crossover relief/1(pR)
  Flow direction/3(pL) -> Crossover relief/2(pL)
  pump limits/1 -> Flow direction/2(Q)

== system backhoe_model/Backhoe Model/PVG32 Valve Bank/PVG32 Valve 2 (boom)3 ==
  note: flow to load
  note: flow through relief valve
  QP : Inport  Port=1  PortWidth=-1  SampleTime=-1  DataType=auto
  pT : Inport  Port=2  PortWidth=-1  SampleTime=-1  DataType=auto
  Us : Inport  Port=3  PortWidth=-1  SampleTime=-1  DataType=auto
  pA : Inport  Port=4  PortWidth=-1  SampleTime=-1  DataType=auto
  pB : Inport  Port=5  PortWidth=-1  SampleTime=-1  DataType=auto
  Crossover relief : Subsystem  Orientation=left
  Dead Zone : DeadZone  LowerValue=-.5  UpperValue=.5
  Flow direction : Subsystem
  Input Averaging : Subsystem
  Product : Product  Inputs=2  SaturateOnIntegerOverflow=on
  SS gain : Subsystem
  Sum : Sum  Inputs=|+-  SaturateOnIntegerOverflow=on
  Terminator : Terminator
  Terminator2 : Terminator
  Time  Delay : TransportDelay  DelayTime=td  InitialInput=0  BufferSize=2048
  Valve dynamics : TransferFcn  Numerator=num  Denominator=den
  pump limits : Saturate  UpperLimit=QP  LowerLimit=-QP
  QA : Outport  Port=1
  QB : Outport  Port=2
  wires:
  pB/1 -> Flow direction/4(pB)
  pA/1 -> Flow direction/3(pA)
  pT/1 -> Terminator2/1
  Time  Delay/1 -> Valve dynamics/1
  Us/1 -> Dead Zone/1
  Dead Zone/1 -> Time  Delay/1, Flow direction/1(Us), Input Averaging/1(Us)
  Valve dynamics/1 -> Product/1
  Input Averaging/1(Ubar) -> SS gain/1(Ubar)
  SS gain/1(Kv) -> Product/2
  Product/1 -> Sum/1, Crossover relief/3(Q)
  Crossover relief/1(Qrelief) -> Sum/2
  QP/1 -> Terminator/1
  Sum/1 -> pump limits/1
  Flow direction/1(QA) -> QA/1
  Flow direction/2(QB) -> QB/1
  Flow direction/4(pR) -> Crossover relief/1(pR)
  Flow direction/3(pL) -> Crossover relief/2(pL)
  pump limits/1 -> Flow direction/2(Q)

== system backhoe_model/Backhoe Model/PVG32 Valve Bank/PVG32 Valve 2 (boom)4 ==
  note: flow to load
  note: flow through relief valve
  QP : Inport  Port=1  PortWidth=-1  SampleTime=-1  DataType=auto
  pT : Inport  Port=2  PortWidth=-1  SampleTime=-1  DataType=auto
  Us : Inport  Port=3  PortWidth=-1  SampleTime=-1  DataType=auto
  pA : Inport  Port=4  PortWidth=-1  SampleTime=-1  DataType=auto
  pB : Inport  Port=5  PortWidth=-1  SampleTime=-1  DataType=auto
  Crossover relief : Subsystem  Orientation=left
  Dead Zone : DeadZone  LowerValue=-.5  UpperValue=.5
  Flow direction : Subsystem
  Input Averaging : Subsystem
  Product : Product  Inputs=2  SaturateOnIntegerOverflow=on
  SS gain : Subsystem
  Sum : Sum  Inputs=|+-  SaturateOnIntegerOverflow=on
  Terminator : Terminator
  Terminator2 : Terminator
  Time  Delay : TransportDelay  DelayTime=td  InitialInput=0  BufferSize=2048
  Valve dynamics : TransferFcn  Numerator=num  Denominator=den
  pump limits : Saturate  UpperLimit=QP  LowerLimit=-QP
  QA : Outport  Port=1
  QB : Outport  Port=2
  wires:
  pB/1 -> Flow direction/4(pB)
  pA/1 -> Flow direction/3(pA)
  pT/1 -> Terminator2/1
  Time  Delay/1 -> Valve dynamics/1
  Us/1 -> Dead Zone/1
  Dead Zone/1 -> Time  Delay/1, Flow direction/1(Us), Input Averaging/1(Us)
  Valve dynamics/1 -> Product/1
  Input Averaging/1(Ubar) -> SS gain/1(Ubar)
  SS gain/1(Kv) -> Product/2
  Product/1 -> Sum/1, Crossover relief/3(Q)
  Crossover relief/1(Qrelief) -> Sum/2
  QP/1 -> Terminator/1
  Sum/1 -> pump limits/1
  Flow direction/1(QA) -> QA/1
  Flow direction/2(QB) -> QB/1
  Flow direction/4(pR) -> Crossover relief/1(pR)
  Flow direction/3(pL) -> Crossover relief/2(pL)
  pump limits/1 -> Flow direction/2(Q)

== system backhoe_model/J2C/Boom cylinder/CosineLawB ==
  TA1B : Inport  Port=1  PortWidth=-1  SampleTime=-1  DataType=auto
  Constant : Constant  Value=2
  Product : Product  Inputs=4  SaturateOnIntegerOverflow=on
  Sum2 : Sum  Inputs=-++  SaturateOnIntegerOverflow=on
  cosine : Trigonometry  Operator=cos  OutputSignalType=auto
  rA : Constant  Value=R1A
  rB : Constant  Value=R1B
  sqr : Fcn  Expr=u^2
  sqr1 : Fcn  Expr=u^2
  sqrt : Fcn  Expr=sqrt(u)
  yc3 : Outport  Port=1
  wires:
  rA/1 -> sqr/1, Product/2
  sqr1/1 -> Sum2/3
  Constant/1 -> Product/1
  sqr/1 -> Sum2/2
  Product/1 -> Sum2/1
  Sum2/1 -> sqrt/1
  TA1B/1 -> cosine/1
  sqrt/1 -> yc3/1
  rB/1 -> sqr1/1, [rB]
  [rB] -> Product/3
  cosine/1 -> Product/4

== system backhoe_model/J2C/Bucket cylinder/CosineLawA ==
  r1 : Inport  Port=1  PortWidth=-1  SampleTime=-1  DataType=auto
  r2 : Inport  Port=2  PortWidth=-1  SampleTime=-1  DataType=auto
  r3 : Inport  Port=3  PortWidth=-1  SampleTime=-1  DataType=auto
  Fcn1 : Fcn  Expr=u^2
  Fcn2 : Fcn  Expr=u^2
  Fcn3 : Fcn  Expr=u^2
  Gain : Gain  Gain=2  SaturateOnIntegerOverflow=on
  Product : Product  Inputs=2  SaturateOnIntegerOverflow=on
  Product1 : Product  Inputs=*/  SaturateOnIntegerOverflow=on
  Sum : Sum  Inputs=++-  SaturateOnIntegerOverflow=on
  Trigonometric Function : Trigonometry  Operator=acos  OutputSignalType=auto
  T3FG : Outport  Port=1
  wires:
  r3/1 -> Fcn3/1
  Fcn1/1 -> Sum/1
  Fcn2/1 -> Sum/2
  Fcn3/1 -> Sum/3
  r2/1 -> Fcn2/1, Product/1
  r1/1 -> Fcn1/1, Product/2
  Product/1 -> Gain/1
  Sum/1 -> Product1/1
  Gain/1 -> Product1/2
  Product1/1 -> Trigonometric Function/1
  Trigonometric Function/1 -> T3FG/1

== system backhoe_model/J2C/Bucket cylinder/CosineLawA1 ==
  r1 : Inport  Port=1  PortWidth=-1  SampleTime=-1  DataType=auto
  r2 : Inport  Port=2  PortWidth=-1  SampleTime=-1  DataType=auto
  r3 : Inport  Port=3  PortWidth=-1  SampleTime=-1  DataType=auto
  Fcn1 : Fcn  Expr=u^2
  Fcn2 : Fcn  Expr=u^2
  Fcn3 : Fcn  Expr=u^2
  Gain : Gain  Gain=2  SaturateOnIntegerOverflow=on
  Product : Product  Inputs=2  SaturateOnIntegerOverflow=on
  Product1 : Product  Inputs=*/  SaturateOnIntegerOverflow=on
  Sum : Sum  Inputs=++-  SaturateOnIntegerOverflow=on
  Trigonometric Function : Trigonometry  Operator=acos  OutputSignalType=auto
  THFG : Outport  Port=1
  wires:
  r3/1 -> Fcn3/1
  Fcn1/1 -> Sum/1
  Fcn2/1 -> Sum/2
  Fcn3/1 -> Sum/3
  r2/1 -> Fcn2/1, Product/1
  r1/1 -> Fcn1/1, Product/2
  Product/1 -> Gain/1
  Sum/1 -> Product1/1
  Gain/1 -> Product1/2
  Product1/1 -> Trigonometric Function/1
  Trigonometric Function/1 -> THFG/1

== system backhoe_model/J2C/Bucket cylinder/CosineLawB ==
  TG3F : Inport  Port=1  PortWidth=-1  SampleTime=-1  DataType=auto
  Constant : Constant  Value=2
  Product : Product  Inputs=4  SaturateOnIntegerOverflow=on
  Sum2 : Sum  Inputs=-++  SaturateOnIntegerOverflow=on
  cosine : Trigonometry  Operator=cos  OutputSignalType=auto
  rA : Constant  Value=R3F
  rB : Constant  Value=R3G
  sqr : Fcn  Expr=u^2
  sqr1 : Fcn  Expr=u^2
  sqrt : Fcn  Expr=sqrt(u)
  rFG : Outport  Port=1
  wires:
  rA/1 -> sqr/1, Product/2
  sqr1/1 -> Sum2/3
  Constant/1 -> Product/1
  sqr/1 -> Sum2/2
  Product/1 -> Sum2/1
  Sum2/1 -> sqrt/1
  TG3F/1 -> cosine/1
  sqrt/1 -> rFG/1
  rB/1 -> sqr1/1, [rB]
  [rB] -> Product/3
  cosine/1 -> Product/4

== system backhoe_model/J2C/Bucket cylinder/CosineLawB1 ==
  TEFH : Inport  Port=1  PortWidth=-1  SampleTime=-1  DataType=auto
  Constant : Constant  Value=2
  Product : Product  Inputs=4  SaturateOnIntegerOverflow=on
  Sum2 : Sum  Inputs=-++  SaturateOnIntegerOverflow=on
  cosine : Trigonometry  Operator=cos  OutputSignalType=auto
  rA : Constant  Value=REF
  rB : Constant  Value=RFH
  sqr : Fcn  Expr=u^2
  sqr1 : Fcn  Expr=u^2
  sqrt : Fcn  Expr=sqrt(u)
  yc5 : Outport  Port=1
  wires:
  rA/1 -> sqr/1, Product/2
  sqr1/1 -> Sum2/3
  Constant/1 -> Product/1
  sqr/1 -> Sum2/2
  Product/1 -> Sum2/1
  Sum2/1 -> sqrt/1
  TEFH/1 -> cosine/1
  sqrt/1 -> yc5/1
  rB/1 -> sqr1/1, [rB]
  cosine/1 -> Product/4
  [rB] -> Product/3

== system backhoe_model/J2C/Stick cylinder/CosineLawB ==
  TC2D : Inport  Port=1  PortWidth=-1  SampleTime=-1  DataType=auto
  Constant : Constant  Value=2
  Product : Product  Inputs=4  SaturateOnIntegerOverflow=on
  Sum2 : Sum  Inputs=-++  SaturateOnIntegerOverflow=on
  cosine : Trigonometry  Operator=cos  OutputSignalType=auto
  rA : Constant  Value=R2C
  rB : Constant  Value=R2D
  sqr : Fcn  Expr=u^2
  sqr1 : Fcn  Expr=u^2
  sqrt : Fcn  Expr=sqrt(u)
  yc4 : Outport  Port=1
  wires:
  rA/1 -> sqr/1, Product/2
  sqr1/1 -> Sum2/3
  Constant/1 -> Product/1
  sqr/1 -> Sum2/2
  Product/1 -> Sum2/1
  Sum2/1 -> sqrt/1
  TC2D/1 -> cosine/1
  sqrt/1 -> yc4/1
  rB/1 -> sqr1/1, [rB]
  cosine/1 -> Product/4
  [rB] -> Product/3

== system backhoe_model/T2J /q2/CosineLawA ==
  r1 : Inport  Port=1  PortWidth=-1  SampleTime=-1  DataType=auto
  r2 : Inport  Port=2  PortWidth=-1  SampleTime=-1  DataType=auto
  r3 : Inport  Port=3  PortWidth=-1  SampleTime=-1  DataType=auto
  Fcn1 : Fcn  Expr=u^2
  Fcn2 : Fcn  Expr=u^2
  Fcn3 : Fcn  Expr=u^2
  Gain : Gain  Gain=2  SaturateOnIntegerOverflow=on
  Product : Product  Inputs=2  SaturateOnIntegerOverflow=on
  Product1 : Product  Inputs=*/  SaturateOnIntegerOverflow=on
  Sum : Sum  Inputs=++-  SaturateOnIntegerOverflow=on
  Trigonometric Function : Trigonometry  Operator=acos  OutputSignalType=auto
  theta : Outport  Port=1
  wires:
  r3/1 -> Fcn3/1
  Fcn1/1 -> Sum/1
  Fcn2/1 -> Sum/2
  Fcn3/1 -> Sum/3
  r2/1 -> Fcn2/1, Product/1
  r1/1 -> Fcn1/1, Product/2
  Product/1 -> Gain/1
  Sum/1 -> Product1/1
  Gain/1 -> Product1/2
  Product1/1 -> Trigonometric Function/1
  Trigonometric Function/1 -> theta/1

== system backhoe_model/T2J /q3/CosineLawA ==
  r1 : Inport  Port=1  PortWidth=-1  SampleTime=-1  DataType=auto
  r2 : Inport  Port=2  PortWidth=-1  SampleTime=-1  DataType=auto
  r3 : Inport  Port=3  PortWidth=-1  SampleTime=-1  DataType=auto
  Fcn1 : Fcn  Expr=u^2
  Fcn2 : Fcn  Expr=u^2
  Fcn3 : Fcn  Expr=u^2
  Gain : Gain  Gain=2  SaturateOnIntegerOverflow=on
  Product : Product  Inputs=2  SaturateOnIntegerOverflow=on
  Product1 : Product  Inputs=*/  SaturateOnIntegerOverflow=on
  Sum : Sum  Inputs=++-  SaturateOnIntegerOverflow=on
  Trigonometric Function : Trigonometry  Operator=acos  OutputSignalType=auto
  theta : Outport  Port=1
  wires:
  r3/1 -> Fcn3/1
  Fcn1/1 -> Sum/1
  Fcn2/1 -> Sum/2
  r2/1 -> Fcn2/1, Product/1
  r1/1 -> Fcn1/1, Product/2
  Product/1 -> Gain/1
  Sum/1 -> Product1/1
  Gain/1 -> Product1/2
  Product1/1 -> Trigonometric Function/1
  Trigonometric Function/1 -> theta/1
  Fcn3/1 -> Sum/3

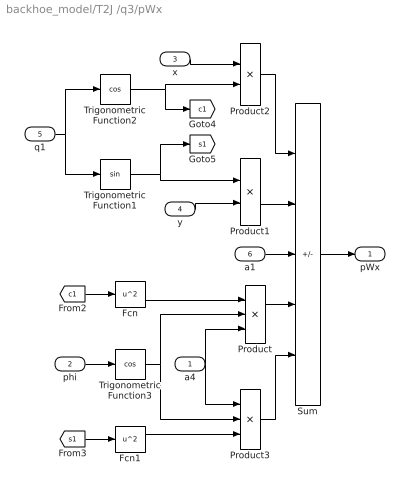
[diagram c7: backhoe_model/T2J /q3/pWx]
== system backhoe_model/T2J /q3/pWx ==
  a4 : Inport  Port=1  PortWidth=-1  SampleTime=-1  DataType=auto
  phi : Inport  Port=2  PortWidth=-1  SampleTime=-1  DataType=auto
  x : Inport  Port=3  PortWidth=-1  SampleTime=-1  DataType=auto
  y : Inport  Port=4  PortWidth=-1  SampleTime=-1  DataType=auto
  q1 : Inport  Port=5  PortWidth=-1  SampleTime=-1  DataType=auto
  a1 : Inport  Port=6  PortWidth=-1  SampleTime=-1  DataType=auto
  Fcn : Fcn  Expr=u^2
  Fcn1 : Fcn  Expr=u^2
  Product : Product  Inputs=3  SaturateOnIntegerOverflow=on
  Product1 : Product  Inputs=2  SaturateOnIntegerOverflow=on
  Product2 : Product  Inputs=2  SaturateOnIntegerOverflow=on
  Product3 : Product  Inputs=3  SaturateOnIntegerOverflow=on
  Sum : Sum  Inputs=++-++  SaturateOnIntegerOverflow=on
  Trigonometric Function1 : Trigonometry  Operator=sin  OutputSignalType=auto
  Trigonometric Function2 : Trigonometry  Operator=cos  OutputSignalType=auto
  Trigonometric Function3 : Trigonometry  Operator=cos  OutputSignalType=auto
  pWx : Outport  Port=1
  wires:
  Product2/1 -> Sum/1
  Product1/1 -> Sum/2
  x/1 -> Product2/1
  Sum/1 -> pWx/1
  q1/1 -> Trigonometric Function2/1, Trigonometric Function1/1
  y/1 -> Product1/2
  Trigonometric Function1/1 -> Product1/1, [s1]
  Trigonometric Function2/1 -> Product2/2, [c1]
  [c1] -> Fcn/1
  Fcn/1 -> Product/1
  a4/1 -> Product3/1, Product/3
  Trigonometric Function3/1 -> Product/2, Product3/2
  [s1] -> Fcn1/1
  phi/1 -> Trigonometric Function3/1
  Fcn1/1 -> Product3/3
  a1/1 -> Sum/3
  Product/1 -> Sum/4
  Product3/1 -> Sum/5

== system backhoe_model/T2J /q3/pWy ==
  z : Inport  Port=1  PortWidth=-1  SampleTime=-1  DataType=auto
  phi : Inport  Port=2  PortWidth=-1  SampleTime=-1  DataType=auto
  a4 : Inport  Port=3  PortWidth=-1  SampleTime=-1  DataType=auto
  Product : Product  Inputs=2  SaturateOnIntegerOverflow=on
  Sum : Sum  Inputs=|++  SaturateOnIntegerOverflow=on
  Trigonometric Function : Trigonometry  Operator=sin  OutputSignalType=auto
  pWy : Outport  Port=1
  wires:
  Trigonometric Function/1 -> Product/2
  a4/1 -> Product/1
  Product/1 -> Sum/1
  Sum/1 -> pWy/1
  phi/1 -> Trigonometric Function/1
  z/1 -> Sum/2

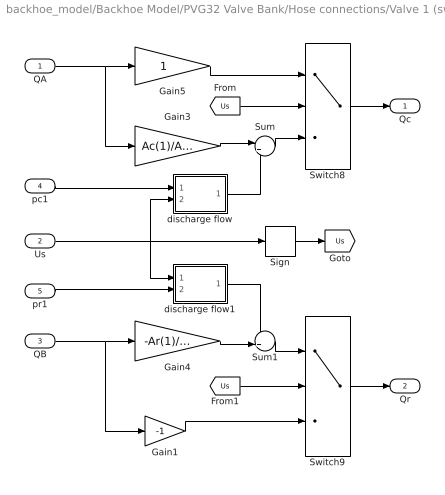
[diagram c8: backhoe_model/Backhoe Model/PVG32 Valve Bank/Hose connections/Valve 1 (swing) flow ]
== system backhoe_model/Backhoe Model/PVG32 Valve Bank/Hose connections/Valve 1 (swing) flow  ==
  QA : Inport  Port=1  PortWidth=-1  SampleTime=-1  DataType=auto
  Us : Inport  Port=2  PortWidth=-1  SampleTime=-1  DataType=auto
  QB : Inport  Port=3  PortWidth=-1  SampleTime=-1  DataType=auto
  pc1 : Inport  Port=4  PortWidth=-1  SampleTime=-1  DataType=auto
  pr1 : Inport  Port=5  PortWidth=-1  SampleTime=-1  DataType=auto
  Gain1 : Gain  Gain=-1  SaturateOnIntegerOverflow=on
  Gain3 : Gain  Gain=Ac(1)/Ar(1)  SaturateOnIntegerOverflow=on
  Gain4 : Gain  Gain=-Ar(1)/Ac(1)  SaturateOnIntegerOverflow=on
  Gain5 : Gain  Gain=1  SaturateOnIntegerOverflow=on
  Sign : Signum
  Sum : Sum  Inputs=|+-  SaturateOnIntegerOverflow=on
  Sum1 : Sum  Inputs=-+|  SaturateOnIntegerOverflow=on
  Switch8 : Switch  Threshold=0
  Switch9 : Switch  Threshold=0
  discharge flow : Subsystem
  discharge flow1 : Subsystem
  Qc : Outport  Port=1
  Qr : Outport  Port=2
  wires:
  [Us] -> Switch8/2
  Gain5/1 -> Switch8/1
  QA/1 -> Gain3/1, Gain5/1
  Switch8/1 -> Qc/1
  Sum/1 -> Switch8/3
  Gain3/1 -> Sum/1
  [Us] -> Switch9/2
  Gain1/1 -> Switch9/3
  QB/1 -> Gain4/1, Gain1/1
  Switch9/1 -> Qr/1
  Sum1/1 -> Switch9/1
  Gain4/1 -> Sum1/2
  pr1/1 -> discharge flow1/2(p)
  discharge flow1/1(Qd) -> Sum1/1
  Us/1 -> discharge flow1/1(Us), discharge flow/2(Us), Sign/1
  pc1/1 -> discharge flow/1(p)
  discharge flow/1(Qd) -> Sum/2
  Sign/1 -> [Us]

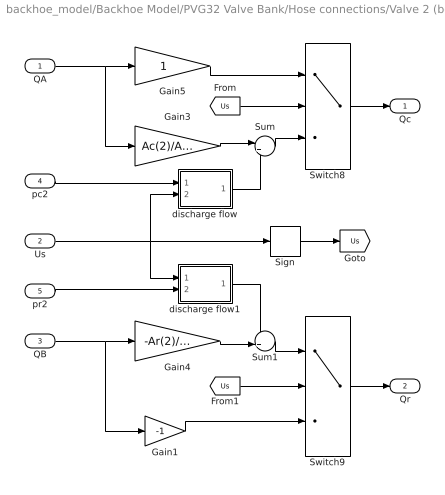
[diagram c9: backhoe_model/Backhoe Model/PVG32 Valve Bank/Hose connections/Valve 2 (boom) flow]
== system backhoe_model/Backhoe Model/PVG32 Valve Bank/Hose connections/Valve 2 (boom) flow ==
  QA : Inport  Port=1  PortWidth=-1  SampleTime=-1  DataType=auto
  Us : Inport  Port=2  PortWidth=-1  SampleTime=-1  DataType=auto
  QB : Inport  Port=3  PortWidth=-1  SampleTime=-1  DataType=auto
  pc2 : Inport  Port=4  PortWidth=-1  SampleTime=-1  DataType=auto
  pr2 : Inport  Port=5  PortWidth=-1  SampleTime=-1  DataType=auto
  Gain1 : Gain  Gain=-1  SaturateOnIntegerOverflow=on
  Gain3 : Gain  Gain=Ac(2)/Ar(2)  SaturateOnIntegerOverflow=on
  Gain4 : Gain  Gain=-Ar(2)/Ac(2)  SaturateOnIntegerOverflow=on
  Gain5 : Gain  Gain=1  SaturateOnIntegerOverflow=on
  Sign : Signum
  Sum : Sum  Inputs=|+-  SaturateOnIntegerOverflow=on
  Sum1 : Sum  Inputs=-+|  SaturateOnIntegerOverflow=on
  Switch8 : Switch  Threshold=0
  Switch9 : Switch  Threshold=0
  discharge flow : Subsystem
  discharge flow1 : Subsystem
  Qc : Outport  Port=1
  Qr : Outport  Port=2
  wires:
  [Us] -> Switch8/2
  Gain5/1 -> Switch8/1
  QA/1 -> Gain3/1, Gain5/1
  Switch8/1 -> Qc/1
  Sum/1 -> Switch8/3
  Gain3/1 -> Sum/1
  [Us] -> Switch9/2
  Gain1/1 -> Switch9/3
  QB/1 -> Gain4/1, Gain1/1
  Switch9/1 -> Qr/1
  Sum1/1 -> Switch9/1
  Gain4/1 -> Sum1/2
  discharge flow/1(Qd) -> Sum/2
  discharge flow1/1(Qd) -> Sum1/1
  pr2/1 -> discharge flow1/2(p)
  pc2/1 -> discharge flow/1(p)
  Us/1 -> discharge flow/2(Us), discharge flow1/1(Us), Sign/1
  Sign/1 -> [Us]
